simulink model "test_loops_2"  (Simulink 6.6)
settings: Solver=ode45  StartTime=0.0  StopTime=10.0  RelTol=1e-3
undefined symbols (not defined in the file or in its folder): data1, test_loops_2
libraries: sltpda x4

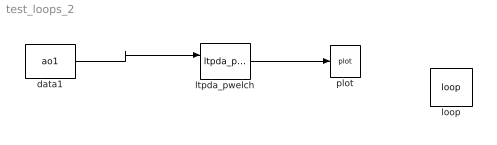
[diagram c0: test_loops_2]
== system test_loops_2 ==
  data1 : sltpda/Sources/ao1  Tag=ao  Description=Creates an Analysis object from a file.  SystemSampleTime=-1  fname=data1.txt
  loop : sltpda/Parameters/loop  SystemSampleTime=-1  block=test_loops_2/data1  blockHandle=270.0030517578125  key=fname  vals=data1.txt data2.txt data3.txt  loopon=on  level=1
  ltpda_pwelch : sltpda/Signal Processing blocks/Frequency domain/ltpda_pwelch  Tag=ltpda_pwelch  Description=Makes a spectral density estimate by calling ltpda_pwlech.  SystemSampleTime=-1
  plot : sltpda/Sinks/plot  Tag=plot  Description=Plot an analysis object.  SystemSampleTime=-1  xscale=linear  yscale=linear
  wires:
  data1/1 -> ltpda_pwelch/1
  ltpda_pwelch/1 -> plot/1
